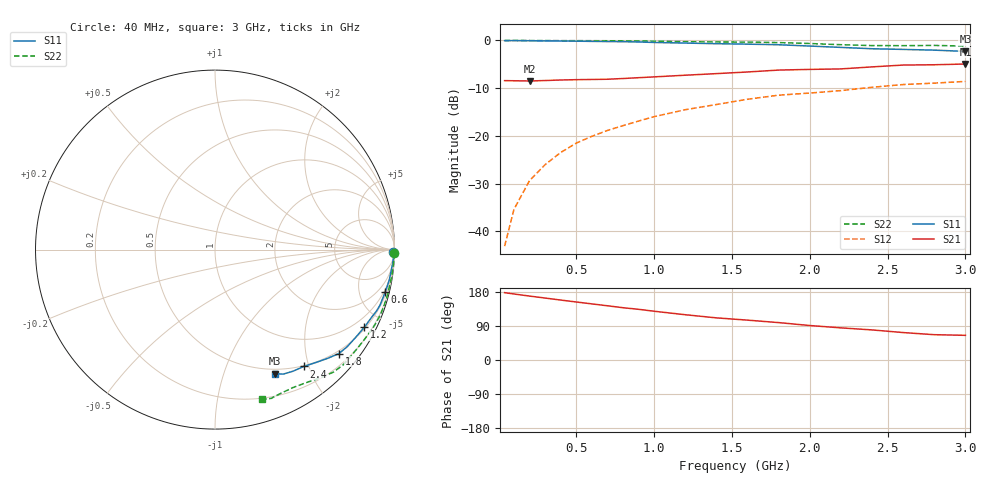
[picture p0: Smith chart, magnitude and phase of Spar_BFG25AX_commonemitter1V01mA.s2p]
! Filename:  BFG25AXA.S2P  Version:  2.0
! NXP part #: BFG25A/X  Date: May 1990
! Bias condition: Vce=1.0V, Ic=0.1mA
#  MHz  S  MA  R  50
! Freq  S11  S21  S12  S22  !GUM [dB]
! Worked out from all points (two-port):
!   21 points, 40 MHz to 3 GHz, reference 50 ohm
!   highest |S21| = -4.94 dB at 3 GHz (marker M1); lowest = -8.5 dB at 200 MHz (marker M2)
!   |S21| within 3 dB of the highest: 821.4 MHz to end of sweep
!   lowest |S11| = -2.3 dB at 3 GHz (marker M3), VSWR 7.58, Z = 22.3 - j74.9 ohm
!   |S11| at or under -10 dB: nowhere
!   |S22| runs from -1.2 to 0.0 dB; largest |S21 - S12| = 0.38
!   S11 on the Smith chart (normalised r, x): 40 MHz: open; 600 MHz: 0.77, -8.01; 1.2 GHz: 0.56, -4.03; 1.8 GHz: 0.44, -2.69; 2.4 GHz: 0.49, -1.92; 3 GHz: 0.45, -1.50
40  0.994 -0.8  0.379 177.7  0.007 88.0  0.999 -1.1
100  0.996 -2.4  0.378 174.2  0.017 88.5  0.999 -2.8
200  0.992 -4.8  0.376 168.7  0.034 85.4  0.997 -5.6
300  0.988 -7.1  0.38 163.5  0.05 83.7  0.996 -8.4
400  0.986 -9.5  0.385 158.2  0.067 81.5  0.994 -11.1
500  0.982 -11.7  0.388 153.1  0.084 79.8  0.994 -13.9
600  0.977 -14.1  0.39 148.1  0.099 78.3  0.993 -16.6
700  0.973 -16.3  0.392 143.1  0.114 76.7  0.992 -19.1
800  0.97 -18.6  0.399 138.0  0.128 75.1  0.99 -21.7
900  0.963 -20.7  0.407 133.8  0.143 73.3  0.986 -24.2
1000  0.952 -23.0  0.415 128.7  0.159 71.3  0.982 -26.7
1200  0.938 -27.4  0.432 119.5  0.188 66.8  0.97 -31.8
1400  0.924 -31.9  0.449 111.2  0.213 63.5  0.963 -36.8
1600  0.914 -36.3  0.467 105.2  0.242 60.9  0.961 -41.8
1800  0.901 -40.0  0.489 98.7  0.267 57.3  0.949 -46.0
2000  0.873 -43.9  0.497 91.0  0.281 53.5  0.928 -50.1
2200  0.845 -48.0  0.503 84.8  0.298 50.2  0.902 -54.8
2400  0.818 -52.7  0.528 79.4  0.323 45.9  0.883 -60.4
2600  0.805 -57.3  0.552 72.4  0.345 41.4  0.881 -65.6
2800  0.791 -61.3  0.556 66.8  0.357 38.9  0.886 -69.4
3000  0.767 -64.3  0.566 65.1  0.372 38.9  0.873 -72.7
